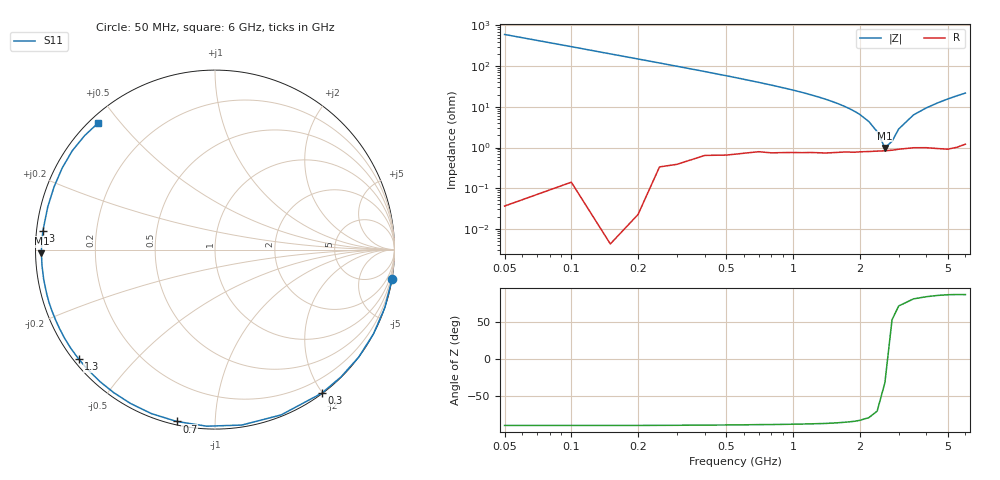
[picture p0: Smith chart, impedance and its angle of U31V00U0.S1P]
! SIEMENS Discrete & RF Semiconductors
! BBY53-02W
! Si Tuning Diode in SCD-80
! VR = 1 V
! S-Parameters:  September  1997
# GHz  S  MA  R  50
!  f  S11
! GHz  MAG  ANG
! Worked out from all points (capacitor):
!   34 points, 50 MHz to 6 GHz, reference 50 ohm
!   read as one part to ground: C = 5.27 pF near 50 MHz
!   lowest |Z| = 982 mohm at 2.6 GHz (marker M1)
!   series resonance near 2.663 GHz, so ESL is about 680 pH
!   S11 on the Smith chart (normalised r, x): 50 MHz: 0, -12; 300 MHz: 0.01, -1.99; 700 MHz: 0.02, -0.80; 1.3 GHz: 0.01, -0.35; 3 GHz: 0.02, +0.05; 6 GHz: 0.02, +0.44
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0.05  1 -9.5
0.1  0.9999 -18.8
0.15  1 -28.0
0.2  0.9999 -36.8
0.25  0.998 -45.3
0.3  0.9969 -53.4
0.4  0.992 -68.2
0.5  0.989 -81.3
0.6  0.985 -92.7
0.7  0.9809 -102.6
0.8  0.98 -111.2
0.9  0.978 -118.8
1  0.9765 -125.3
1.1  0.9755 -131.2
1.2  0.9743 -136.6
1.3  0.9738 -141.3
1.4  0.9736 -145.6
1.6  0.9716 -153.2
1.9  0.9705 -162.5
2.2  0.9688 -170.2
2.4  0.9679 -174.7
2.6  0.9673 -178.8
3  0.9644 173.8
3.5  0.9618 165.7
4  0.9624 158.7
5  0.9673 145.3
5.5  0.9649 138.9
6  0.9602 132.9
